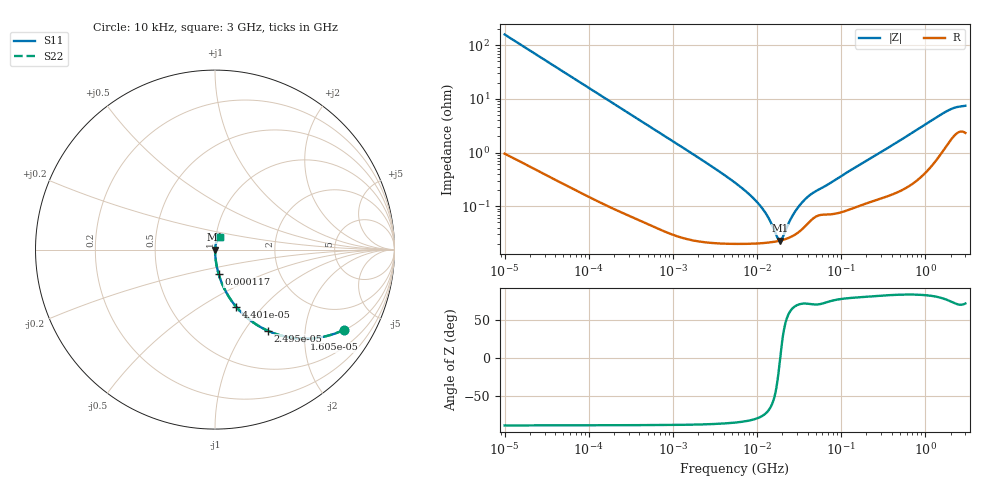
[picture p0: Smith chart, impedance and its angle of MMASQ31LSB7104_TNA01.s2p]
! MMASQ31LSB7104_TNA01  S-PARAMETER MODEL  ( Standard Model )
! Model Generated by TAIYO YUDEN Corporation (http://www.ty-top.com)
! Version 1.0
! TAIYO YUDEN Control No. 220601
! Copyright(c) 2013 TAIYO YUDEN CO.,LTD. All Rights Reserved.
! Product Description (link to TY-COMPAS)
! https://ds.yuden.co.jp/TYCOMPAS/or/detail?pn=MMASQ31LSB7104KTNA01&u=M
! Products Name : Multilayer Ceramic Capacitors
! Characteristics :
!  Capacitance : 0.1 [uF] , Rated Voltage : 250 [V] , TCC : X7R
!  Case Size : 3.2 x 1.6 / 0.126 x 0.063 [mm/inch] , Thickness : 1.6 / 0.063 [mm/inch]
!  (Conditions: Temperature = 25 [degC] , DC Bias Voltage = 0 [V])
! External Node Assignments :
!  1  o---| |---o  2
! GND o---------o GND
! Frequency Range : 10kHz  -  3GHz  [ 401 STEP ]
# MHZ S RI R 50
! Freq[MHz].  S11 Real  S11 Imag  S21 Real  S21 Imag  S12 Real  S12 Imag  S22 Real  S22 Imag
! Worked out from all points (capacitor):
!   401 points, 10 kHz to 3 GHz, reference 50 ohm
!   read as one part in series: C = 99.7 nF near 10.65 kHz
!   lowest |Z| = 22.8 mohm at 18.73 MHz (marker M1)
!   series resonance near 18.87 MHz, so ESL is about 710 pH
!   S11 on the Smith chart (normalised r, x): 10 kHz: 1.02, -3.19; 16.05 kHz: 1.01, -1.99; 24.95 kHz: 1.01, -1.28; 44.01 kHz: 1.01, -0.73; 117 kHz: 1.00, -0.28; 3 GHz: 1.05, +0.14
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0.01  0.7167 -0.4476  0.2833 0.4476  0.2833 0.4476  0.7167 -0.4476
0.016047  0.4979 -0.4967  0.5021 0.4967  0.5021 0.4967  0.4979 -0.4967
0.024951  0.293 -0.4516  0.707 0.4516  0.707 0.4516  0.293 -0.4516
0.044011  0.1193 -0.3203  0.8807 0.3203  0.8807 0.3203  0.1193 -0.3203
0.082683  0.0381 -0.187  0.9619 0.187  0.9619 0.187  0.0381 -0.187
0.11696  0.0199 -0.135  0.9801 0.135  0.9801 0.135  0.0199 -0.135
0.683653  0.000941 -0.0238  0.9991 0.0238  0.9991 0.0238  0.000941 -0.0238
5.477226  0.000206 -0.00274  0.9998 0.00274  0.9998 0.00274  0.000206 -0.00274
8.252149  0.000202 -0.00161  0.9998 0.00161  0.9998 0.00161  0.000202 -0.00161
11.31085  0.000205 -0.000931  0.9998 0.000931  0.9998 0.000931  0.000205 -0.000931
14.10408  0.000211 -0.000516  0.9998 0.000516  0.9998 0.000516  0.000211 -0.000516
17.5871  0.000223 -0.000124  0.9998 0.000124  0.9998 0.000124  0.000223 -0.000124
18.73182  0.000228 -1.31e-05  0.9998 1.31e-05  0.9998 1.31e-05  0.000228 -1.31e-05
19.95104  0.000234 9.75e-05  0.9998 -9.75e-05  0.9998 -9.75e-05  0.000234 9.75e-05
24.87798  0.000265 0.000492  0.9997 -0.000492  0.9997 -0.000492  0.000265 0.000492
29.12589  0.000304 0.000789  0.9997 -0.000789  0.9997 -0.000789  0.000304 0.000789
36.31858  0.000406 0.00122  0.9996 -0.00122  0.9996 -0.00122  0.000406 0.00122
45.28751  0.000573 0.00164  0.9994 -0.00164  0.9994 -0.00164  0.000573 0.00164
374.4521  0.00173 0.0126  0.9983 -0.0126  0.9983 -0.0126  0.00173 0.0126
1755.269  0.0157 0.0549  0.9843 -0.0549  0.9843 -0.0549  0.0157 0.0549
2258.843  0.025 0.0628  0.975 -0.0628  0.975 -0.0628  0.025 0.0628
3000  0.0274 0.0674  0.9726 -0.0674  0.9726 -0.0674  0.0274 0.0674
